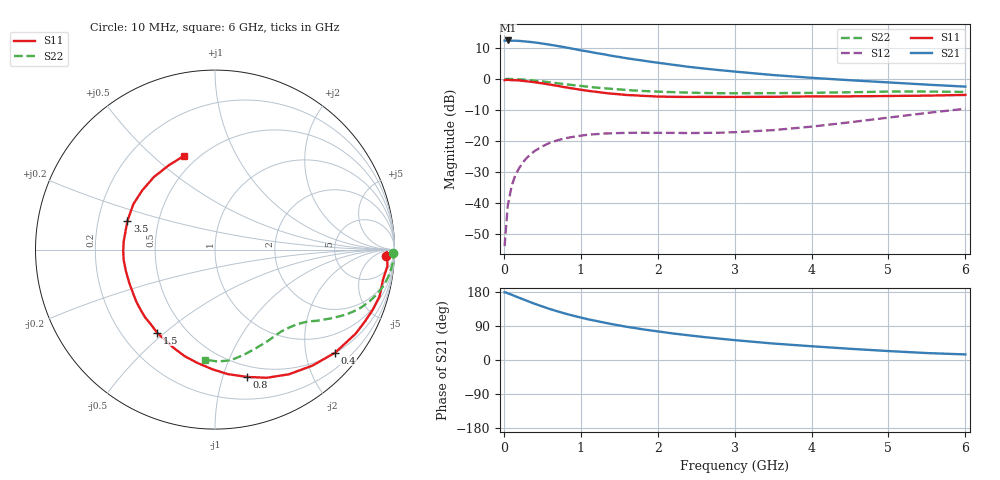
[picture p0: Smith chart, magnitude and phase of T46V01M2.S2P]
! Infineon Technologies  Discrete & RF Semiconductors
! BFR182T
! Si NPN RF Bipolar Junction Transistor in SC75
! VCE = 6 V  IC = 1.2 mA
! Common Emitter S-Parameters:  October  1999
# GHz  S  MA  R  50
!  f  S11  S21  S12  S22
! GHz  MAG  ANG  MAG  ANG  MAG  ANG  MAG  ANG
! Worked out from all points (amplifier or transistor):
!   36 points, 10 MHz to 6 GHz, reference 50 ohm
!   highest |S21| = 12.4 dB at 50 MHz (marker M1)
!   |S21| within 3 dB of that: start of sweep to 961.4 MHz
!   unconditionally stable (mu >= 1): 2.33 GHz to 4.546 GHz
!   at 250 MHz: K = 0.10, MSG = 19.5 dB, |S12| = -26.9 dB
!   at 1.4 GHz: K = 0.62, MSG = 12.5 dB, |S12| = -17.6 dB
!   at 6 GHz: K = 0.83, MSG = 3.6 dB, |S12| = -9.6 dB
!   S11 on the Smith chart (normalised r, x): 10 MHz: 27, -19; 400 MHz: 0.51, -2.62; 800 MHz: 0.39, -1.20; 1.5 GHz: 0.35, -0.47; 3.5 GHz: 0.33, +0.14; 6 GHz: 0.42, +0.64
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0.01  0.9518 -2.0  4.137 178.6  0.002 86.6  0.9911 -1.2
0.02  0.9577 -0.8  4.115 178.8  0.0029 93.3  0.9901 -0.7
0.05  0.9651 -5.4  4.161 176.0  0.0088 90.3  0.9958 -2.1
0.1  0.951 -10.1  4.129 172.4  0.0184 83.5  0.994 -4.1
0.15  0.9531 -15.9  4.126 168.1  0.0282 80.9  0.9872 -6.2
0.25  0.927 -25.4  4.041 160.2  0.0452 74.9  0.9715 -10.1
0.4  0.882 -40.6  3.868 148.4  0.0685 66.6  0.9356 -15.5
0.5  0.8445 -49.9  3.715 141.3  0.0815 61.7  0.9078 -18.5
0.6  0.8078 -59.3  3.55 134.4  0.0932 57.3  0.8783 -21.4
0.7  0.7702 -68.0  3.383 128.3  0.1023 53.3  0.8485 -23.8
0.8  0.7313 -75.9  3.227 122.4  0.1102 49.9  0.8196 -26.0
0.9  0.6971 -84.2  3.05 117.0  0.116 46.5  0.7915 -27.9
1.1  0.6389 -98.9  2.753 107.1  0.1258 41.5  0.7449 -31.1
1.3  0.5949 -112.5  2.49 98.9  0.1313 37.9  0.7054 -33.9
1.5  0.564 -124.9  2.255 91.2  0.1336 35.5  0.6757 -36.1
1.8  0.5319 -141.8  1.978 81.1  0.1353 33.3  0.6379 -39.6
2.2  0.5125 -158.9  1.687 70.0  0.1344 33.8  0.6103 -43.9
2.8  0.5115 -179.4  1.384 56.5  0.1352 38.9  0.5865 -51.4
3.5  0.5133 162.1  1.152 43.5  0.1488 48.4  0.5882 -60.4
4.5  0.5226 140.9  0.95 29.6  0.1992 58.3  0.6075 -74.5
5.5  0.5358 118.6  0.807 18.3  0.2816 59.4  0.6236 -88.7
6  0.5506 108.1  0.749 14.7  0.3296 57.0  0.6154 -95.3
